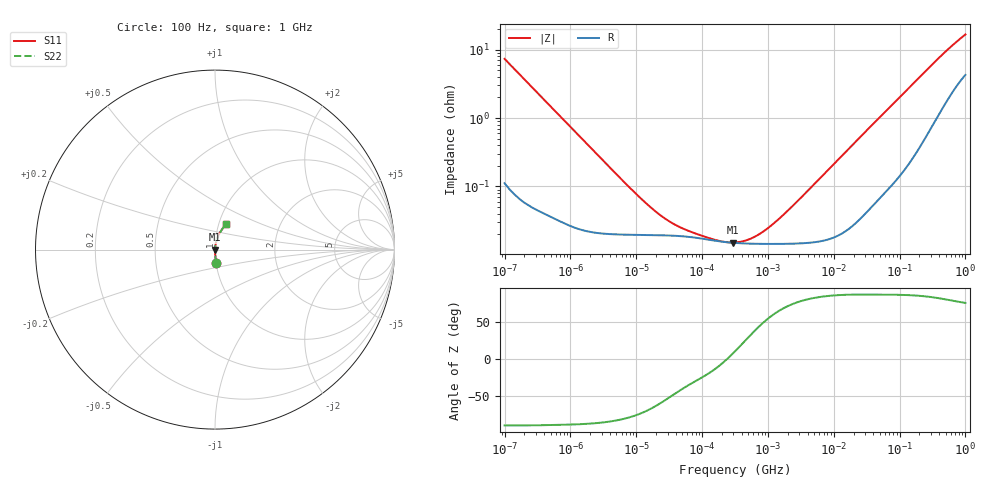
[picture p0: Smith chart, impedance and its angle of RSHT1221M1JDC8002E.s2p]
! RSHT1221M1JDC8002E  S-PARAMETER MODEL  (General Type)
! Model Generated by ELNA Corporation (http://www.ty-top.com)
! Version 1.0
! ELNA Control No.240229
! Copyright (c) 2024 ELNA CO.,LTD. All Rights Reserved.
! Products Name : CONDUCTIVE POLYMER HYBRID ALUMINUM ELECTROLYTIC CAPACITORS
! Characteristics :
!  Capacitance  :  220uF  ,  Rated voltage  :  6.3V
!  Operating Temp. Range  :  -55 to +105 degC  ,  Endurance  :  10000hr at 105 degC
!  Dimension D  :  6.3mm  ,  Dimension L  :  5.8mm
! Frequency Range : 100Hz - 1GHz
! External Node Assignments :
!  1  o---| |---o  2
# MHz S RI R 50
!Freq[MHz].  S11 Real  S11 Imag  S21 Real  S21 Imag  S12 Real  S12 Imag  S22 Real  S22 Imag
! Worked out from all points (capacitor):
!   401 points, 100 Hz to 1 GHz, reference 50 ohm
!   read as one part in series: C = 217 uF near 108 Hz
!   lowest |Z| = 15.1 mohm at 291.7 kHz (marker M1)
!   series resonance near 240.5 kHz, so ESL is about 2 nH
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0.0001  0.00643 -0.0727  0.9936 0.0727  0.9936 0.0727  0.00643 -0.0727
0.000113  0.00515 -0.0645  0.9949 0.0645  0.9949 0.0645  0.00515 -0.0645
0.000309  0.00102 -0.0237  0.999 0.0237  0.999 0.0237  0.00102 -0.0237
0.001488  0.000256 -0.005  0.9997 0.005  0.9997 0.005  0.000256 -0.005
0.00912  0.000197 -0.00082  0.9998 0.00082  0.9998 0.00082  0.000197 -0.00082
0.014791  0.000195 -0.000508  0.9998 0.000508  0.9998 0.000508  0.000195 -0.000508
0.022131  0.000194 -0.000342  0.9998 0.000342  0.9998 0.000342  0.000194 -0.000342
0.037368  0.00019 -0.000207  0.9998 0.000207  0.9998 0.000207  0.00019 -0.000207
0.06569  0.000182 -0.000122  0.9998 0.000122  0.9998 0.000122  0.000182 -0.000122
0.165959  0.00016 -3.39e-05  0.9998 3.39e-05  0.9998 3.39e-05  0.00016 -3.39e-05
0.291743  0.00015 1.88e-05  0.9998 -1.88e-05  0.9998 -1.88e-05  0.00015 1.88e-05
0.316228  0.000149 2.7e-05  0.9999 -2.7e-05  0.9999 -2.7e-05  0.000149 2.7e-05
0.419276  0.000147 5.8e-05  0.9999 -5.8e-05  0.9999 -5.8e-05  0.000147 5.8e-05
0.533949  0.000146 8.87e-05  0.9999 -8.87e-05  0.9999 -8.87e-05  0.000146 8.87e-05
0.901571  0.000144 0.000176  0.9999 -0.000176  0.9999 -0.000176  0.000144 0.000176
1.717908  0.000145 0.000356  0.9999 -0.000356  0.9999 -0.000356  0.000145 0.000356
4.704354  0.000152 0.000993  0.9998 -0.000993  0.9998 -0.000993  0.000152 0.000993
69.9842  0.00115 0.0141  0.9989 -0.0141  0.9989 -0.0141  0.00115 0.0141
184.0772  0.00451 0.036  0.9955 -0.036  0.9955 -0.036  0.00451 0.036
395.8221  0.0165 0.0728  0.9835 -0.0728  0.9835 -0.0728  0.0165 0.0728
695.825  0.0398 0.1137  0.9602 -0.1137  0.9602 -0.1137  0.0398 0.1137
1000  0.0632 0.1445  0.9368 -0.1445  0.9368 -0.1445  0.0632 0.1445
